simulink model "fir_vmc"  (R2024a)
settings: Solver=ode45  StartTime=0.0  StopTime=300  RelTol=1e-3  EnableMultiTasking=on
undefined symbols (not defined in the file or in its folder): C, code, Evaluation, ffva1156, gateway_in_config, gateway_out_config, hex2dec, HLS, KCU105, Kintex, netlist, Platform, sysgen, UltraScale, xcku040
libraries: hdlBasic x11, vmcUtilities x1

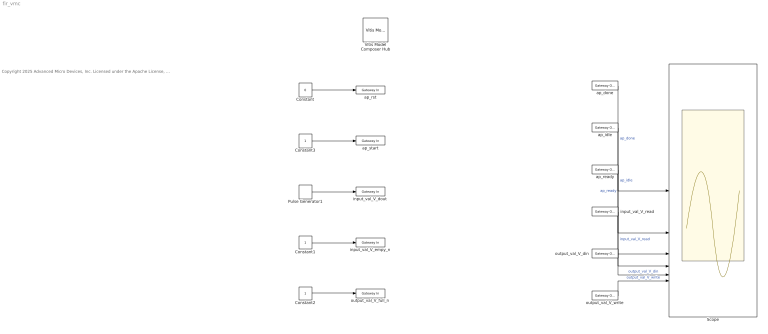
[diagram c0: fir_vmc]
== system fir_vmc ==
  note: Copyright 2025 Advanced Micro Devices, Inc. Licensed under the Apache License, Version 2.0 (the "License"); you may not use this file except in compliance with the License. You may obtain a copy of the License at http://www.apache.org/licenses/LICENSE-2.0 Unless required by applicable law or agreed to in writing, software distributed under the License is distributed on an "AS IS" BASIS, WITHOUT WARRANTIES OR CONDITIONS OF ANY KIND, either express or implied. See the License for the specific language governing permissions and limitations under the License.
  Constant : Constant  Value=0  SampleTime=1
  Constant1 : Constant  SampleTime=1
  Constant2 : Constant  SampleTime=1
  Constant3 : Constant  SampleTime=1
  Pulse Generator1 : DiscretePulseGenerator  Period=10000  PhaseDelay=25
  Scope : Scope  NumInputPorts=6
  Vitis Model Composer Hub : vmcUtilities/Vitis Model Composer Hub  Tag=genX  CodeGeneration=off  SubsystemName=<enter or select subsystem name>  StartColumn=1  NumberOfColumns=1  TargetDirectory=./code  exportDesign=off  analyzeDesign=off  validateDesignOnHw=off  ExportType=HLS C++ code  IpVendor=xilinx.com  IpLibrary=hls  IpVersion=1.0  IpHWLanguage=Verilog  AieCompilerOptions={}  AieSimulatorOptions={}  CreateTestbench=off  TestbenchStackSize=10  RunRtlSim=off  RunCSim=off  RunAieSim=off  AieSimTimeout=50000  RunAieSimProfiling=off  LaunchVitisAnalyzer=off  PlotOutput=off  RunX86Sim=off  X86SimTimeout=10  GenHwImage=off  GenLibadfXo=off  GenHwValidationCode=off  PlatformType=Not Specified  HwSystemType=Baremetal  HwValidationTarget=hw  ProjDevice=Kintex-UltraScale KCU105 Evaluation Platform (xcku040-ffva1156-2-e)  ProjDevicePart=xcku040-ffva1156-2-e  SamplePeriod=-1  ClockFrequency=200  DataPathParallelism=1  xilinxfamily=kintexu  part=xcku040  speed=-2-e  package=ffva1156  directory=./netlist  testbench=off  incr_netlist=off  synthesis_tool=Vivado  clock_wrapper=Clock Enables  dbl_ovrd=According to Block Masks  dcm_input_clock_period=10  sysclk_period=10  simulink_period=1  eval_field=0  LogFileName=''  NThreads=4
  ap_done : hdlBasic/Gateway Out  inherit_from_input=off  hdl_port=on  rows=1  columns=1  UseAsDAC=off  DACChannel='1'  interface=None  automatic_assignment=on  address_offset=hex2dec('00')  intf_name=''  intf_description=''  timing_constraint=None  locs_specified=off  LOCs={}  io_standard={}  XmcBlockStatus=1  maskContainerNames=group4  block_type=gatewayout  block_config=sysgen:gateway_out_config  block_width_w=590  block_height_w=620  block_width=620  block_height=750
  ap_idle : hdlBasic/Gateway Out  inherit_from_input=off  hdl_port=on  rows=1  columns=1  UseAsDAC=off  DACChannel='1'  interface=None  automatic_assignment=on  address_offset=hex2dec('00')  intf_name=''  intf_description=''  timing_constraint=None  locs_specified=off  LOCs={}  io_standard={}  XmcBlockStatus=1  maskContainerNames=group4  block_type=gatewayout  block_config=sysgen:gateway_out_config  block_width_w=590  block_height_w=620  block_width=620  block_height=750
  ap_ready : hdlBasic/Gateway Out  inherit_from_input=off  hdl_port=on  rows=1  columns=1  UseAsDAC=off  DACChannel='1'  interface=None  automatic_assignment=on  address_offset=hex2dec('00')  intf_name=''  intf_description=''  timing_constraint=None  locs_specified=off  LOCs={}  io_standard={}  XmcBlockStatus=1  maskContainerNames=group4  block_type=gatewayout  block_config=sysgen:gateway_out_config  block_width_w=590  block_height_w=620  block_width=620  block_height=750
  ap_rst : hdlBasic/Gateway In  gui_display_data_type=Boolean  arith_type=Boolean  n_bits=16  bin_pt=14  preci_type=Single  exp_width=8  frac_width=24  rows=1  columns=1  quantization="Round  (unbiased: +/- Inf)"  overflow=Saturate  period=1  UseAsADC=off  ADCChannel='1'  interface=None  automatic_assignment=on  address_offset=hex2dec('00')  intf_name=''  intf_description=''  default_value=0  timing_constraint=None  locs_specified=off  LOCs={}  io_standard={}  inherit_from_input=off  hdl_port=on  XmcBlockStatus=1  maskContainerNames=group4  block_type=gatewayin  block_config=sysgen:gateway_in_config  block_width_w=590  block_height_w=620  block_width=640  block_height=850
  ap_start : hdlBasic/Gateway In  gui_display_data_type=Boolean  arith_type=Boolean  n_bits=16  bin_pt=14  preci_type=Single  exp_width=8  frac_width=24  rows=1  columns=1  quantization="Round  (unbiased: +/- Inf)"  overflow=Saturate  period=1  UseAsADC=off  ADCChannel='1'  interface=None  automatic_assignment=on  address_offset=hex2dec('00')  intf_name=''  intf_description=''  default_value=0  timing_constraint=None  locs_specified=off  LOCs={}  io_standard={}  inherit_from_input=off  hdl_port=on  XmcBlockStatus=1  maskContainerNames=group4  block_type=gatewayin  block_config=sysgen:gateway_in_config  block_width_w=590  block_height_w=620  block_width=640  block_height=850
  input_val_V_dout : hdlBasic/Gateway In  gui_display_data_type=Fixed-point  arith_type=Signed (2's comp)  n_bits=32  bin_pt=0  preci_type=Single  exp_width=8  frac_width=24  rows=1  columns=1  quantization="Round  (unbiased: +/- Inf)"  overflow=Saturate  period=1  UseAsADC=off  ADCChannel='1'  interface=None  automatic_assignment=on  address_offset=hex2dec('00')  intf_name=''  intf_description=''  default_value=0  timing_constraint=None  locs_specified=off  LOCs={}  io_standard={}  inherit_from_input=off  hdl_port=on  XmcBlockStatus=1  maskContainerNames=group4  block_type=gatewayin  block_config=sysgen:gateway_in_config  block_width_w=590  block_height_w=620  block_width=640  block_height=850
  input_val_V_empy_n : hdlBasic/Gateway In  gui_display_data_type=Boolean  arith_type=Boolean  n_bits=16  bin_pt=14  preci_type=Single  exp_width=8  frac_width=24  rows=1  columns=1  quantization="Round  (unbiased: +/- Inf)"  overflow=Saturate  period=1  UseAsADC=off  ADCChannel='1'  interface=None  automatic_assignment=on  address_offset=hex2dec('00')  intf_name=''  intf_description=''  default_value=0  timing_constraint=None  locs_specified=off  LOCs={}  io_standard={}  inherit_from_input=off  hdl_port=on  XmcBlockStatus=1  maskContainerNames=group4  block_type=gatewayin  block_config=sysgen:gateway_in_config  block_width_w=590  block_height_w=620  block_width=640  block_height=850
  input_val_V_read : hdlBasic/Gateway Out  inherit_from_input=off  hdl_port=on  rows=1  columns=1  UseAsDAC=off  DACChannel='1'  interface=None  automatic_assignment=on  address_offset=hex2dec('00')  intf_name=''  intf_description=''  timing_constraint=None  locs_specified=off  LOCs={}  io_standard={}  XmcBlockStatus=1  maskContainerNames=group4  block_type=gatewayout  block_config=sysgen:gateway_out_config  block_width_w=590  block_height_w=620  block_width=620  block_height=750
  output_val_V_din : hdlBasic/Gateway Out  inherit_from_input=off  hdl_port=on  rows=1  columns=1  UseAsDAC=off  DACChannel='1'  interface=None  automatic_assignment=on  address_offset=hex2dec('00')  intf_name=''  intf_description=''  timing_constraint=None  locs_specified=off  LOCs={}  io_standard={}  XmcBlockStatus=1  maskContainerNames=group4  block_type=gatewayout  block_config=sysgen:gateway_out_config  block_width_w=590  block_height_w=620  block_width=620  block_height=750
  output_val_V_full_n : hdlBasic/Gateway In  gui_display_data_type=Boolean  arith_type=Boolean  n_bits=16  bin_pt=14  preci_type=Single  exp_width=8  frac_width=24  rows=1  columns=1  quantization="Round  (unbiased: +/- Inf)"  overflow=Saturate  period=1  UseAsADC=off  ADCChannel='1'  interface=None  automatic_assignment=on  address_offset=hex2dec('00')  intf_name=''  intf_description=''  default_value=0  timing_constraint=None  locs_specified=off  LOCs={}  io_standard={}  inherit_from_input=off  hdl_port=on  XmcBlockStatus=1  maskContainerNames=group4  block_type=gatewayin  block_config=sysgen:gateway_in_config  block_width_w=590  block_height_w=620  block_width=640  block_height=850
  output_val_V_write : hdlBasic/Gateway Out  inherit_from_input=off  hdl_port=on  rows=1  columns=1  UseAsDAC=off  DACChannel='1'  interface=None  automatic_assignment=on  address_offset=hex2dec('00')  intf_name=''  intf_description=''  timing_constraint=None  locs_specified=off  LOCs={}  io_standard={}  XmcBlockStatus=1  maskContainerNames=group4  block_type=gatewayout  block_config=sysgen:gateway_out_config  block_width_w=590  block_height_w=620  block_width=620  block_height=750
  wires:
  ? -> ap_done/1
  ? -> ap_idle/1
  ap_done/1 -> Scope/1  "ap_done"
  ap_idle/1 -> Scope/2  "ap_idle"
  ap_ready/1 -> Scope/3  "ap_ready"
  Constant/1 -> ap_rst/1
  Constant3/1 -> ap_start/1
  Constant1/1 -> input_val_V_empy_n/1
  Constant2/1 -> output_val_V_full_n/1
  Pulse Generator1/1 -> input_val_V_dout/1
  ? -> ap_ready/1
  ? -> output_val_V_din/1
  output_val_V_full_n/1 -> ?
  input_val_V_dout/1 -> ?
  input_val_V_empy_n/1 -> ?
  ap_rst/1 -> ?
  ap_start/1 -> ?
  ? -> input_val_V_read/1
  ? -> output_val_V_write/1
  input_val_V_read/1 -> Scope/4  "input_val_V_read"
  output_val_V_din/1 -> Scope/5  "output_val_V_din"
  output_val_V_write/1 -> Scope/6  "output_val_V_write"
